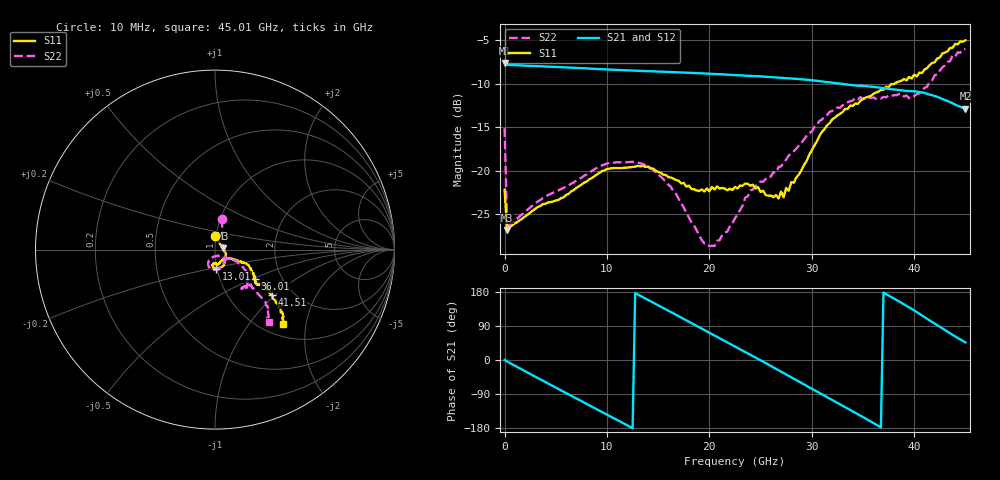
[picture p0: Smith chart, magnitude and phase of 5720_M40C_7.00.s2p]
! Device:  ADRF5720
! Description: 0.5dB LSB GaAs MMIC 6-bit Digital Attenuator
! Frequency:  0.000009 -  40 GHz
! Ports:
!	RF1	= Port 1
!	RF2	= Port 2
! Vdd:  3.3 Volt
! Vss:  -3.3 Volt
! Control:  0/3.3 Volt
! State:  7.00 dB attenuation
! Data:  The device was measured using G-S-G Probes on a matrix board.
!  Data was collected using an calibrated 4 port network analyzer.
!  The reference plane for this measurement is at the launchers.
! Note:  Analog Devices supplies this data as a sample of measured data
!  for this product.  Your particular data for this product may vary.
!  Data was taken at -40 degrees C.
!  Analog Devices reserves the right to change this data at anytime.
# GHZ S DB R 45.0
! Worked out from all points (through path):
!   181 points, 10 MHz to 45.01 GHz, reference 45 ohm
!   highest |S21| = -7.65 dB at 10 MHz (marker M1); lowest = -12.8 dB at 45.01 GHz (marker M2)
!   group delay of S21, straight-line fit = 41.1 ps
!   lowest |S11| = -26.8 dB at 260 MHz (marker M3), VSWR 1.10, Z = 49.2 + j0.638 ohm
!   |S11| at or under -10 dB: start of sweep to 38.08 GHz
!   |S22| runs from -28.7 to -6.0 dB; largest |S21 - S12| = 0.0017
!   S11 on the Smith chart (normalised r, x): 10 MHz: 0.99, +0.15; 13.01 GHz: 0.99, -0.21; 36.01 GHz: 1.46, -0.52; 41.51 GHz: 1.57, -0.95; 45.01 GHz: 1.23, -1.48
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0.01  -22.20 90.8  -7.65 -0.2  -7.67 -0.2  -15.11 77.6
0.26  -26.83 8.2  -7.82 -4.0  -7.84 -4.0  -26.55 6.7
2.26  -25.05 -11.0  -7.93 -33.2  -7.95 -33.2  -24.46 -18.0
4.26  -23.64 -21.4  -8.03 -62.0  -8.05 -62.0  -22.80 -33.0
6.01  -22.80 -35.8  -8.12 -87.2  -8.14 -87.2  -21.80 -47.7
7.76  -21.38 -48.7  -8.22 -112.2  -8.24 -112.2  -20.59 -62.5
10.51  -19.70 -66.9  -8.38 -151.4  -8.41 -151.4  -19.06 -82.6
13.01  -19.44 -86.8  -8.50 173.0  -8.52 172.9  -19.07 -101.6
15.26  -20.24 -96.2  -8.60 140.7  -8.62 140.6  -20.68 -114.4
17.76  -21.83 -97.6  -8.73 104.7  -8.75 104.6  -24.87 -116.0
20.01  -22.37 -92.4  -8.85 72.1  -8.87 72.0  -28.68 -80.9
22.76  -22.04 -85.9  -9.01 32.1  -9.04 32.0  -25.01 -47.2
23.76  -21.51 -81.4  -9.08 17.5  -9.10 17.4  -22.94 -44.3
25.01  -22.44 -69.8  -9.15 -0.8  -9.17 -1.0  -21.25 -37.2
27.26  -23.05 -46.9  -9.33 -34.2  -9.35 -34.4  -19.06 -28.7
30.26  -17.11 -25.3  -9.63 -79.3  -9.66 -79.5  -14.97 -32.3
32.76  -13.46 -26.0  -9.98 -116.9  -10.00 -117.0  -12.75 -40.0
36.01  -11.18 -36.4  -10.35 -166.1  -10.38 -166.3  -11.56 -52.6
37.76  -10.04 -39.1  -10.63 166.5  -10.66 166.3  -11.47 -55.1
39.51  -9.22 -35.2  -10.84 139.1  -10.86 138.9  -11.66 -47.1
41.51  -7.87 -38.6  -11.25 104.5  -11.27 104.3  -9.81 -45.7
45.01  -5.02 -47.6  -12.85 46.4  -12.88 46.2  -6.02 -53.3
